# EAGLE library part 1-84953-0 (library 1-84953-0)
10 way r/a top FFC SMT connector,1mm Source: Datasheet
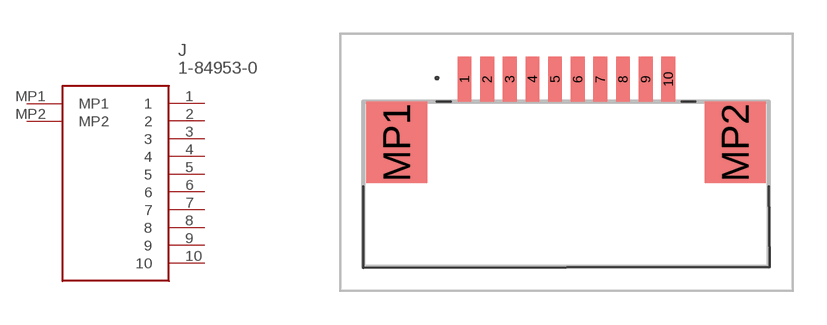
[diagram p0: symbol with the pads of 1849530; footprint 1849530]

Designator prefix J

## 1-84953-0 (Description: 10 way r/a top FFC SMT connector,1mm; Height: 2.74mm; Manufacturer_Name: TE Connectivity; Manufacturer_Part_Number: 1-84953-0; Mouser_Part_Number: 571-1-84953-0; Mouser_Price-Stock: https://www.mouser.co.uk/ProductDetail/TE-Connectivity/1-84953-0?qs=uUkeXfjQ8uROgNfgw1lrfw%3D%3D)  [1849530]
1  1
2  2
3  3
4  4
5  5
6  6
7  7
8  8
9  9
10  10
MP1  MP1
MP2  MP2

## Footprint 1849530 (pad centres in mm)
1-84953-0-1
smd 0.61 x 2: 1 -4.485,4.15; 2 -3.485,4.15; 3 -2.485,4.15; 4 -1.485,4.15; 5 -0.485,4.15; 6 0.515,4.15; 7 1.515,4.15; 8 2.515,4.15; 9 3.515,4.15; 10 4.515,4.15
smd 2.68 x 3.6: MP1 -7.475,1.35; MP2 7.475,1.35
